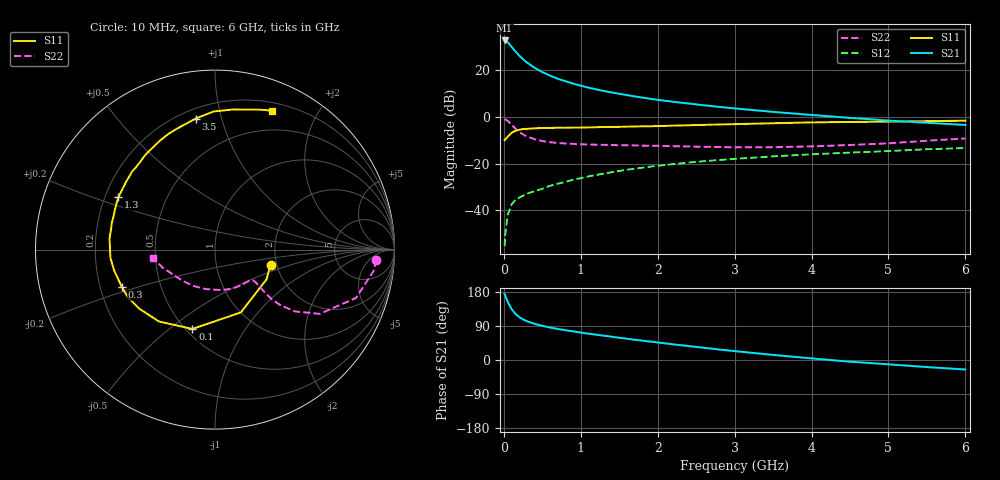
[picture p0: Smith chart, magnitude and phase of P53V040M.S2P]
! SIEMENS Small Signal Semiconductors
! BFP183
! Si NPN RF Bipolar Junction Transistor in SOT143
! VCE = 3 V  IC = 40 mA
! Common Emitter S-Parameters:  March  1996
# GHz  S  MA  R  50
!  f  S11  S21  S12  S22
! GHz  MAG  ANG  MAG  ANG  MAG  ANG  MAG  ANG
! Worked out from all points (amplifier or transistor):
!   36 points, 10 MHz to 6 GHz, reference 50 ohm
!   highest |S21| = 32.9 dB at 10 MHz (marker M1)
!   |S21| within 3 dB of that: start of sweep to 107.4 MHz
!   unconditionally stable (mu >= 1): start of sweep to 11.7 MHz; 433.4 MHz to end of sweep
!   at 250 MHz: K = 0.75, MSG = 29.3 dB, |S12| = -33.8 dB
!   at 1.4 GHz: K = 1.28, MAG = 14.0 dB, |S12| = -23.7 dB
!   at 6 GHz: K = 1.00, MAG = 4.5 dB, |S12| = -13.3 dB
!   S11 on the Smith chart (normalised r, x): 10 MHz: 1.85, -0.35; 100 MHz: 0.54, -0.60; 300 MHz: 0.29, -0.18; 1.3 GHz: 0.25, +0.24; 3.5 GHz: 0.26, +0.83; 6 GHz: 0.28, +1.45
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0.01  0.3205 -15.2  44.09 174.4  0.0017 82.9  0.9009 -3.6
0.02  0.3315 -29.9  43.74 169.2  0.0032 79.4  0.8915 -7.7
0.05  0.3785 -67.6  40.46 153.7  0.008 72.7  0.8304 -18.9
0.1  0.4597 -105.9  32.29 134.6  0.0133 57.1  0.6852 -31.5
0.15  0.5079 -128.0  25.7 121.9  0.0167 51.9  0.5652 -37.6
0.2  0.5343 -141.8  20.85 113.2  0.0187 51.6  0.4808 -40.3
0.25  0.5532 -151.3  17.38 107.0  0.0205 51.8  0.424 -41.2
0.3  0.5593 -158.2  14.87 102.5  0.0227 51.9  0.3834 -40.9
0.4  0.5739 -168.3  11.44 95.4  0.0258 53.6  0.3352 -40.1
0.5  0.5845 -175.5  9.206 90.2  0.029 54.9  0.3063 -39.3
0.6  0.5856 178.6  7.79 85.7  0.0335 57.3  0.2894 -38.8
0.7  0.591 173.8  6.663 81.9  0.0372 58.7  0.2784 -38.8
0.8  0.5898 169.4  5.885 78.6  0.0408 59.2  0.271 -39.2
1.1  0.6008 158.0  4.294 69.4  0.0535 59.4  0.2579 -42.1
1.3  0.6127 151.6  3.629 64.0  0.0613 59.1  0.2535 -45.3
1.7  0.6286 139.1  2.776 53.5  0.0778 56.9  0.2466 -52.7
2.2  0.6557 126.2  2.135 41.4  0.0978 52.7  0.2373 -64.2
2.8  0.6945 112.0  1.654 27.6  0.1201 46.8  0.2281 -81.0
3.5  0.7379 98.4  1.293 13.4  0.1436 40.4  0.2259 -103.4
4.5  0.7863 83.0  0.961 -4.5  0.173 30.7  0.252 -136.7
5.5  0.8177 72.5  0.755 -18.7  0.2043 22.2  0.3111 -161.7
6  0.8367 67.8  0.678 -25.0  0.217 17.3  0.3479 -172.4
